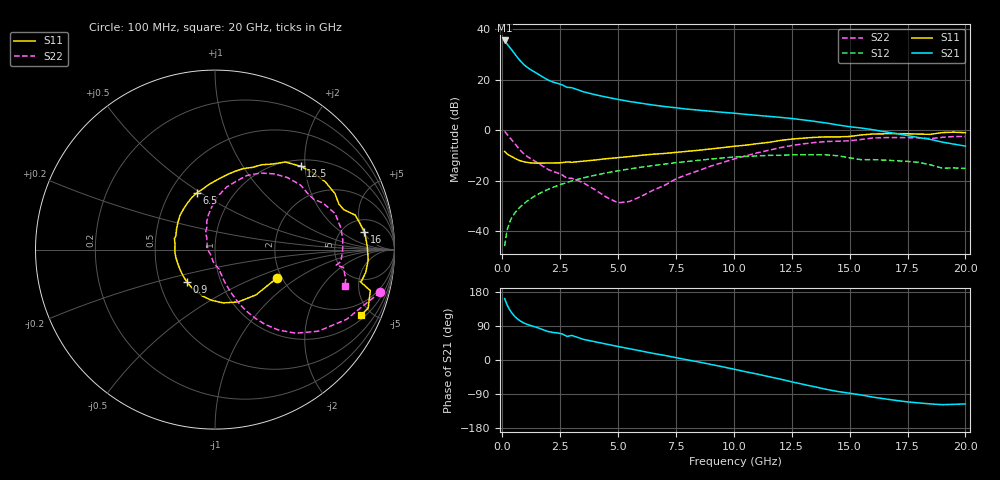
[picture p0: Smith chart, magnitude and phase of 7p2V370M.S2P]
! Infineon Technologies  Discrete & RF Semiconductors
! bfp620
! VCE =  2.3 V,  IC =  70 mA
! Common Emitter S-Parameters:  Sep 2002
# GHz  S  MA  R  50
!  f  S11  S21  S12  S22
! GHz  MAG  ANG  MAG  ANG  MAG  ANG  MAG  ANG
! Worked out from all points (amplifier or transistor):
!   59 points, 100 MHz to 20 GHz, reference 50 ohm
!   highest |S21| = 35.6 dB at 100 MHz (marker M1)
!   |S21| within 3 dB of that: start of sweep to 342.3 MHz
!   unconditionally stable (mu >= 1): 2.123 GHz to 2.324 GHz; 2.467 GHz to 9.841 GHz; 17.19 GHz to end of sweep
!   at 1 GHz: K = 0.88, MSG = 27.1 dB, |S12| = -28.7 dB
!   at 5.5 GHz: K = 1.04, MAG = 12.2 dB, |S12| = -15.4 dB
!   at 20 GHz: K = 1.24, MAG = 1.5 dB, |S12| = -15.2 dB
!   S11 on the Smith chart (normalised r, x): 100 MHz: 1.88, -0.70; 900 MHz: 0.69, -0.26; 6.5 GHz: 0.68, +0.49; 12.5 GHz: 1.14, +1.90; 16 GHz: 7.78, +5.29; 20 GHz: 1.21, -4.34
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0.1  0.3795 -24.7  60.27 161.9  0.005 79.5  0.9508 -14.4
0.2  0.3402 -47.9  51.6 146.5  0.0101 74.1  0.8289 -28.0
0.3  0.3188 -66.2  45.14 134.4  0.0143 71.8  0.7334 -38.3
0.4  0.3006 -81.1  39.52 125.1  0.018 70.3  0.6479 -46.0
0.5  0.2833 -93.8  34.45 117.6  0.0214 69.2  0.5696 -51.8
0.6  0.2678 -105.1  29.97 111.5  0.0246 68.5  0.4999 -56.3
0.7  0.2552 -115.0  26.18 106.4  0.0277 67.9  0.4404 -59.8
0.9  0.2382 -131.1  20.67 98.6  0.0338 67.1  0.3522 -64.6
1.2  0.2256 -147.5  16.14 91.5  0.043 65.8  0.277 -68.4
2  0.2237 -176.6  9.774 74.9  0.0676 60.7  0.1646 -74.6
2.8  0.2342 164.8  7.069 62.3  0.0921 54.1  0.1111 -79.3
3  0.2307 160.9  6.975 64.8  0.0982 52.3  0.1111 -78.5
3.5  0.243 151.9  5.787 54.5  0.1133 47.7  0.0904 -86.2
5  0.2852 128.3  4.077 35.5  0.1567 33.5  0.0362 -134.3
6.5  0.3331 107.3  3.16 17.7  0.1982 19.1  0.064 133.9
7  0.3454 101.0  2.95 12.3  0.2125 14.4  0.0801 124.7
10.5  0.5035 65.5  2.066 -30.9  0.3018 -25.0  0.3079 85.4
12.5  0.6664 44.2  1.705 -57.6  0.3247 -48.6  0.4967 59.2
13.5  0.7216 31.5  1.494 -70.8  0.3251 -61.5  0.5694 44.8
16  0.839 6.9  1.022 -97.9  0.2607 -85.5  0.699 16.7
17  0.8555 -3.8  0.861 -106.7  0.2478 -93.6  0.7142 4.1
20  0.8925 -24.2  0.484 -116.0  0.1746 -103.0  0.7512 -15.8
